FUNCTION "C SPAZZOLATURA" : VOID
TITLE =CICLO SPAZZOLATURA
VERSION : 0.1

BEGIN
NETWORK
TITLE =ATTESA START
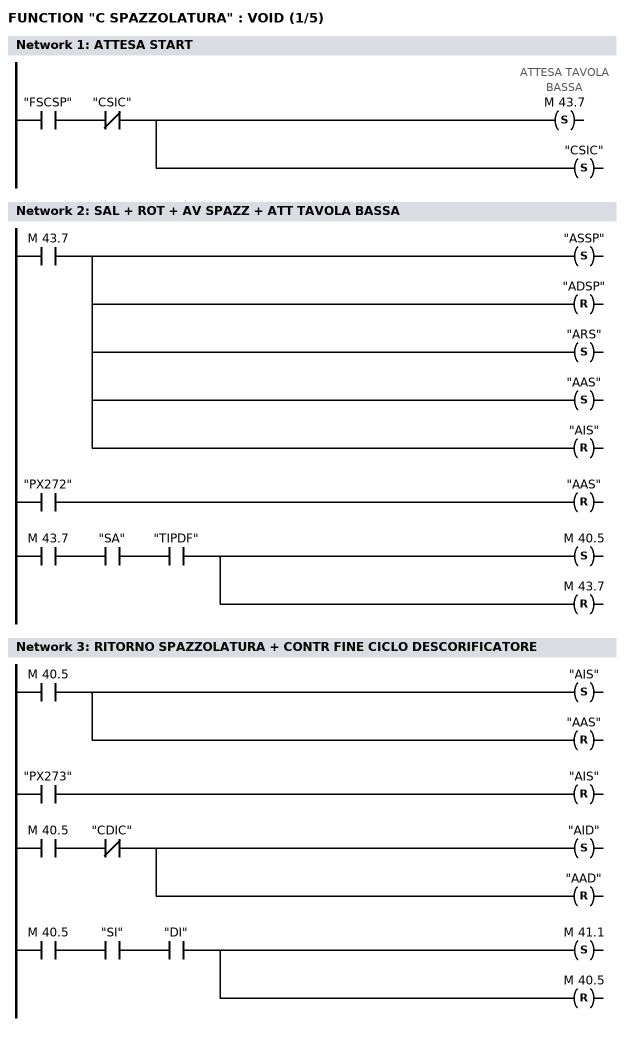
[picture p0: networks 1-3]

      U     "FSCSP";
      UN    "CSIC";
      S     M     43.7; // ATTESA TAVOLA BASSA
      S     "CSIC";
NETWORK
TITLE =SAL + ROT + AV SPAZZ + ATT TAVOLA BASSA

      U     M     43.7;
      S     "ASSP";
      R     "ADSP";
      S     "ARS";
      S     "AAS";
      R     "AIS";

      U     "PX272";
      R     "AAS";

      U     M     43.7;
//U     "SPA"
      U     "SA";
      U     "TIPDF";
      S     M     40.5;
      R     M     43.7;
NETWORK
TITLE =RITORNO SPAZZOLATURA + CONTR FINE CICLO DESCORIFICATORE

      U     M     40.5;
      S     "AIS";
      R     "AAS";

      U     "PX273";
      R     "AIS";

      U     M     40.5;
      UN    "CDIC";
      S     "AID";
      R     "AAD";

      U     M     40.5;
      U     "SI";
//     UN    M     40.6
//      U     M     42.7
      U     "DI";
      S     M     41.1;
      R     M     40.5;
NETWORK
TITLE =SALITA STAGNATURA + SALITA FLUSSAGGIO
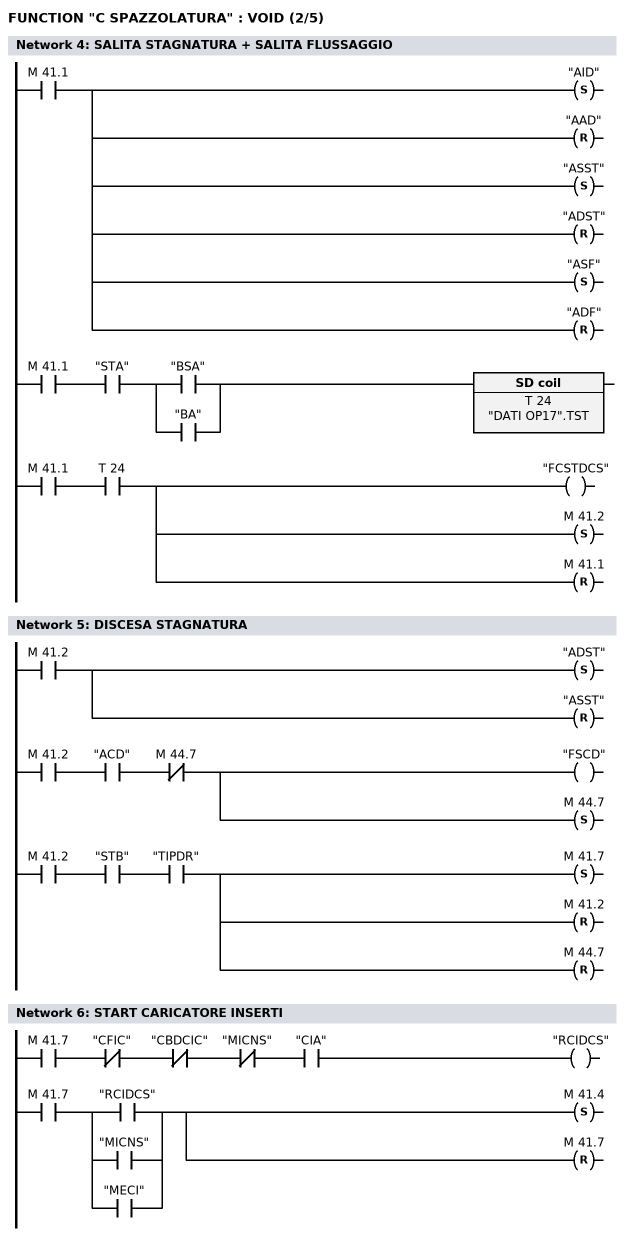
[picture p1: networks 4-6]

      U     M     41.1;
      S     "AID";
      R     "AAD";
      S     "ASST";
      R     "ADST";
      S     "ASF";
      R     "ADF";

      U     M     41.1;
      U     "STA";
      U(    ;
      U     "BSA";
      O     "BA";
      )     ;
      L     "DATI OP17".TST;
      SE    T     24;

      U     M     41.1;
      U     T     24;
      =     "FCSTDCS";
      S     M     41.2;
      R     M     41.1;
NETWORK
TITLE =DISCESA STAGNATURA

      U     M     41.2;
      S     "ADST";
      R     "ASST";

      U     M     41.2;
      U     "ACD";
      UN    M     44.7;
      =     "FSCD";
      S     M     44.7;

      U     M     41.2;
// U     "FLA"
      U     "STB";
      U     "TIPDR";
      S     M     41.7;
      R     M     41.2;
      R     M     44.7;
NETWORK
TITLE =START CARICATORE INSERTI

      U     M     41.7;
      UN    "CFIC";
      UN    "CBDCIC";
      UN    "MICNS";
      U     "CIA";
      =     "RCIDCS";

      U     M     41.7;
      U(    ;
      U     "RCIDCS";
      O     "MICNS";
      O     "MECI";
      )     ;
      S     M     41.4;
      R     M     41.7;
NETWORK
TITLE =
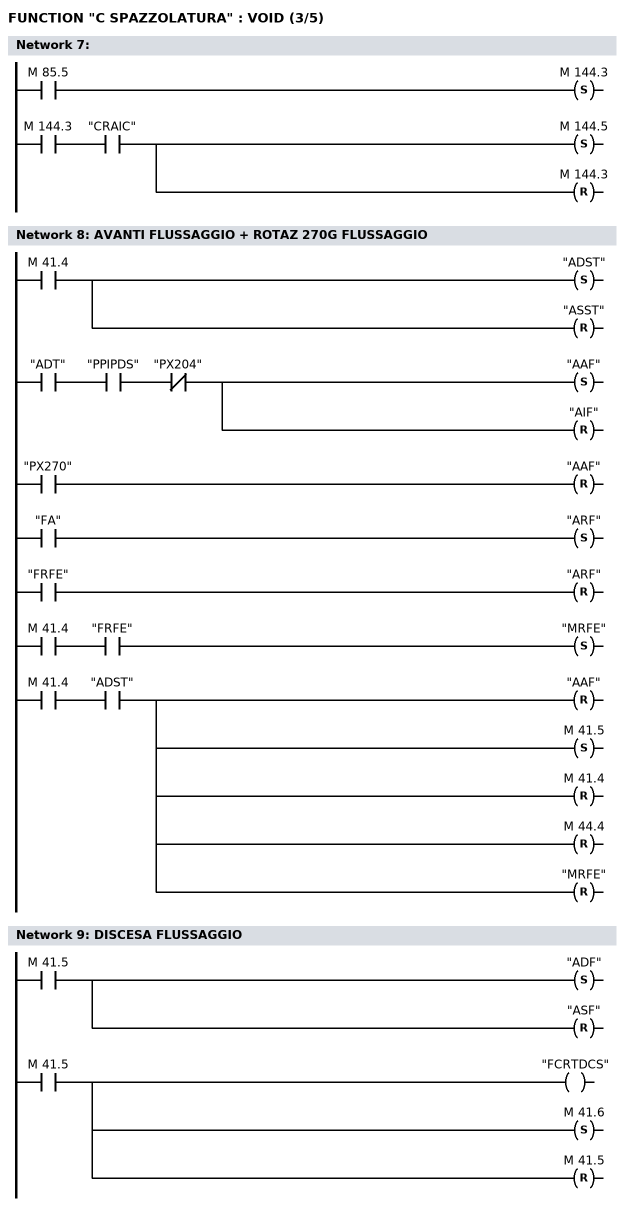
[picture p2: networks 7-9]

      U     M     85.5;
      S     M    144.3;
      U     M    144.3;
      U     "CRAIC";
      S     M    144.5;
      R     M    144.3;
NETWORK
TITLE =AVANTI FLUSSAGGIO + ROTAZ 270G FLUSSAGGIO

      U     M     41.4;
      S     "ADST";
      R     "ASST";
      U     "ADT";
      U     "PPIPDS";
      UN    "PX204";
      S     "AAF";
      R     "AIF";
      U     "PX270";
      R     "AAF";
      U     "FA";
      S     "ARF";
      U     "FRFE";
      R     "ARF";
      U     M     41.4;
      U     "FRFE";
      S     "MRFE";
      U     M     41.4;
      U     "ADST";
      R     "AAF";
      S     M     41.5;
      R     M     41.4;
      R     M     44.4;
      R     "MRFE";

NETWORK
TITLE =DISCESA FLUSSAGGIO

      U     M     41.5;
      S     "ADF";
      R     "ASF";

      U     M     41.5;
// U     "FLB"
      =     "FCRTDCS";
      S     M     41.6;
      R     M     41.5;
NETWORK
TITLE =RITORNO FLUSSAGGIO
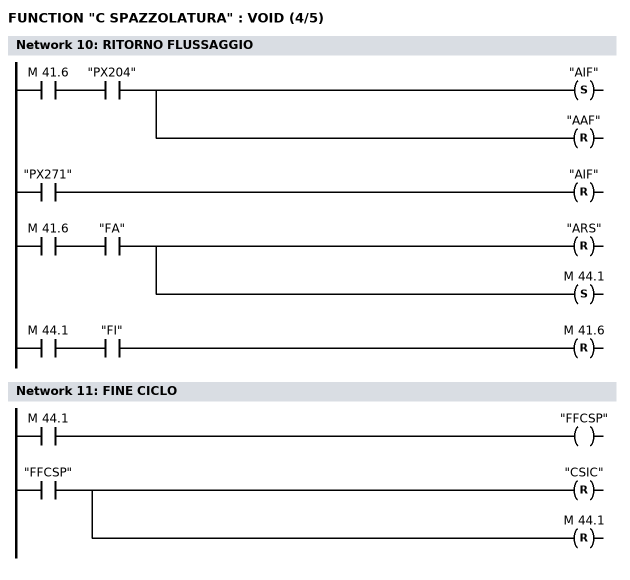
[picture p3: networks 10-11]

      U     M     41.6;
      U     "PX204";
      S     "AIF";
      R     "AAF";
      U     "PX271";
      R     "AIF";
      U     M     41.6;
      U     "FA";
      R     "ARS";
      S     M     44.1;
      U     M     44.1;
      U     "FI";
      R     M     41.6;
NETWORK
TITLE =FINE CICLO

      U     M     44.1;
      =     "FFCSP";

      U     "FFCSP";
      R     "CSIC";
      R     M     44.1;
NETWORK
TITLE =CICLO DESCORIFICATORE
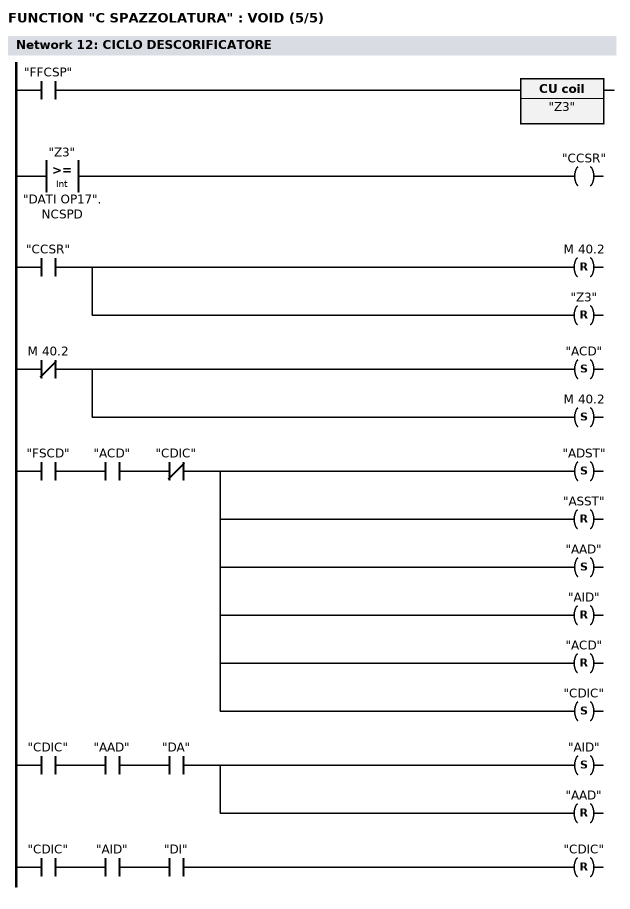
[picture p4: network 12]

      U     "FFCSP";
      ZV    "Z3";

      L     "Z3";
      L     "DATI OP17".NCSPD;
      >=I   ;
      =     "CCSR";

      U     "CCSR";
      R     M     40.2;
      R     "Z3";

      UN    M     40.2;
      S     "ACD";
      S     M     40.2;

      U     "FSCD";
      U     "ACD";
      UN    "CDIC";
      S     "ADST";
      R     "ASST";
      S     "AAD";
      R     "AID";
      R     "ACD";
      S     "CDIC";

      U     "CDIC";
      U     "AAD";
      U     "DA";
      S     "AID";
      R     "AAD";

      U     "CDIC";
      U     "AID";
      U     "DI";
      R     "CDIC";
NETWORK
TITLE =RESET CICLO SPAZZOLATURA

      U     "BRA";
      SPBN  M001;
      L     0;
      T     MB    40;
      T     MB    41;
      T     MB    42;
      T     MB    43;
      T     MB    44;
      SET   ;
      R     "Z3";
M001: NOP   0;
END_FUNCTION

